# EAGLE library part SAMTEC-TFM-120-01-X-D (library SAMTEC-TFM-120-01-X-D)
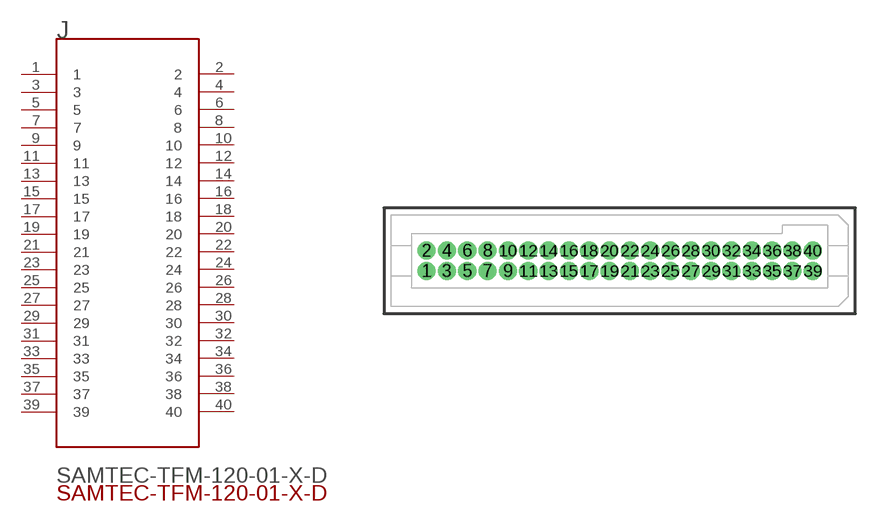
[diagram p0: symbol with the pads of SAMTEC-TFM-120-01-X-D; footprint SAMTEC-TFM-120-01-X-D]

Designator prefix J

## SAMTEC-TFM-120-01-X-DJ (Description: Conn Shrouded Header HDR 40 POS 1.27mm Solder ST Thru-Hole Tube; Digi-Key_Part_Number: SAM10144-ND; Digi-Key_Purchase_URL: https://www.digikey.com/product-detail/en/samtec-inc/TFM-120-01-L-D/SAM10144-ND/6678881?utm_source=snapeda&utm_medium=aggregator&utm_campaign=symbol; MF: Samtec Inc.; MP: TFM-120-01-L-D; Package: None)  [SAMTEC-TFM-120-01-X-D]
1  1  pas
2  2  pas
3  3  pas
4  4  pas
5  5  pas
6  6  pas
7  7  pas
8  8  pas
9  9  pas
10  10  pas
11  11  pas
12  12  pas
13  13  pas
14  14  pas
15  15  pas
16  16  pas
17  17  pas
18  18  pas
19  19  pas
20  20  pas
21  21  pas
22  22  pas
23  23  pas
24  24  pas
25  25  pas
26  26  pas
27  27  pas
28  28  pas
29  29  pas
30  30  pas
31  31  pas
32  32  pas
33  33  pas
34  34  pas
35  35  pas
36  36  pas
37  37  pas
38  38  pas
39  39  pas
40  40  pas

## Footprint SAMTEC-TFM-120-01-X-D (pad centres in mm)
translated Allegro footprint
drill 0.635 pad 1.143: 1 -12.065,-0.635; 2 -12.065,0.635; 3 -10.795,-0.635; 4 -10.795,0.635; 5 -9.525,-0.635; 6 -9.525,0.635; 7 -8.255,-0.635; 8 -8.255,0.635; 9 -6.985,-0.635; 10 -6.985,0.635; 11 -5.715,-0.635; 12 -5.715,0.635; 13 -4.445,-0.635; 14 -4.445,0.635; 15 -3.175,-0.635; 16 -3.175,0.635; 17 -1.905,-0.635; 18 -1.905,0.635; 19 -0.635,-0.635; 20 -0.635,0.635; 21 0.635,-0.635; 22 0.635,0.635; 23 1.905,-0.635; 24 1.905,0.635; 25 3.175,-0.635; 26 3.175,0.635; 27 4.445,-0.635; 28 4.445,0.635; 29 5.715,-0.635; 30 5.715,0.635; 31 6.985,-0.635; 32 6.985,0.635; 33 8.255,-0.635; 34 8.255,0.635; 35 9.525,-0.635; 36 9.525,0.635; 37 10.795,-0.635; 38 10.795,0.635; 39 12.065,-0.635; 40 12.065,0.635

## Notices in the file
This work is licensed under a Creative Commons Attribution-ShareAlike 4.0 International License (CC BY-SA) with Design Exception 1.0
